FUNCTION "FC_CLEAN_ROOM" : VOID
TITLE =FC CLEAN ROOM
{ S7_language := '9(1) Angielski (Stany Zjednoczone)  11.01.2022  09:45:15' }
VERSION : 0.1


VAR_TEMP
  PREHEATING_TIME_SP : S5TIME ;
  FOLLOW_UP_PURGING_ON : BOOL ;
  PREPURING_ON : BOOL ;
  CR_HUM_RELEASE : BOOL ;
  F_UP_PURGING_TIME_SP : S5TIME ;
  H_84CLM82_HUM_SWP : REAL ;
  H_84CLM82_DEHUM_SWP : REAL ;
  T_84CLT81_COOL_SWP : REAL ;
  T_84CLT81_HEAT_SWP : REAL ;
  H_84CLM82_READY_LOW : REAL ;
  H_84CLM82_READY_HIGH : REAL ;
  T_84CLT81_READY_LOW : REAL ;
  T_84CLT81_READY_HIGH : REAL ;
  T_81CLM10_HUM_SP : REAL ;
  T_81CLM10_HUM_AV_REL : REAL ;
  T_81CLM10_HUM_SP_DINT : DINT ;
  T_84CLT32_COOL_SWP : REAL ;
  T_84CLT32_HEAT_SWP : REAL ;
  T_AV_REAL : REAL ;
  T_AV_DINT : DINT ;
END_VAR
BEGIN
NETWORK
TITLE =CLEAN ROOM ON
//********************************************************************************
//
//                         CLEAN ROOM START / STOP
//
//********************************************************************************
//
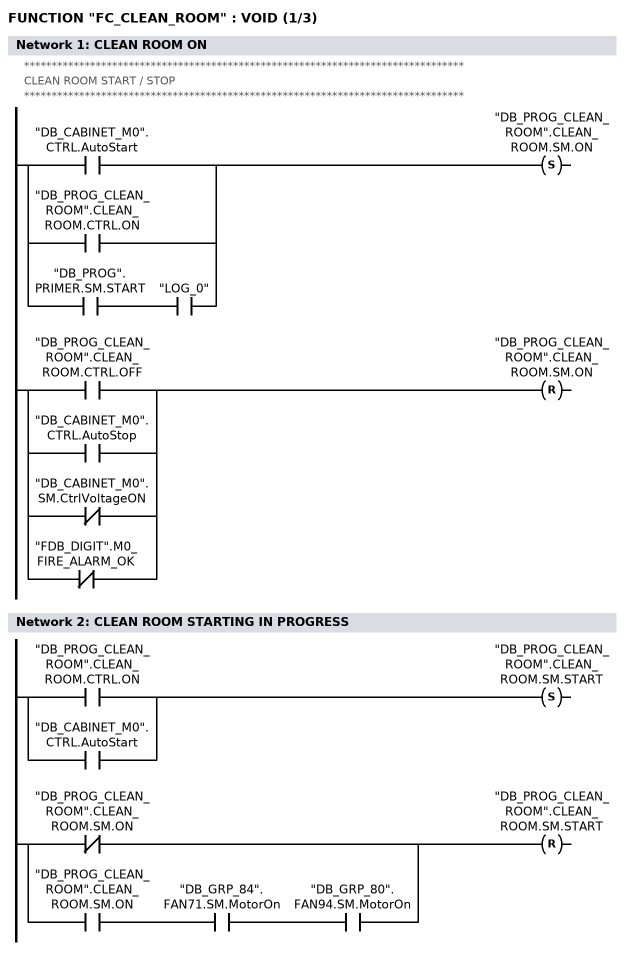
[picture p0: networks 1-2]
      U(    ;
      O     "DB_CABINET_M0".CTRL.AutoStart;
      O     "DB_PROG_CLEAN_ROOM".CLEAN_ROOM.CTRL.ON;
      O     ;
      U     "DB_PROG".PRIMER.SM.START;
      U     "LOG_0";
      )     ;
      S     "DB_PROG_CLEAN_ROOM".CLEAN_ROOM.SM.ON;
      U(    ;
      O     "DB_PROG_CLEAN_ROOM".CLEAN_ROOM.CTRL.OFF;
      O     "DB_CABINET_M0".CTRL.AutoStop;
      ON    "DB_CABINET_M0".SM.CtrlVoltageON;
      ON    "FDB_DIGIT".M0_FIRE_ALARM_OK;
      )     ;
      R     "DB_PROG_CLEAN_ROOM".CLEAN_ROOM.SM.ON;
      NOP   0;
NETWORK
TITLE =CLEAN ROOM STARTING IN PROGRESS

      U(    ;
      O     "DB_PROG_CLEAN_ROOM".CLEAN_ROOM.CTRL.ON;
      O     "DB_CABINET_M0".CTRL.AutoStart;
      )     ;
      S     "DB_PROG_CLEAN_ROOM".CLEAN_ROOM.SM.START;
      U(    ;
      ON    "DB_PROG_CLEAN_ROOM".CLEAN_ROOM.SM.ON;
      O     ;
      U     "DB_PROG_CLEAN_ROOM".CLEAN_ROOM.SM.ON;
      U     "DB_GRP_84".FAN71.SM.MotorOn;
      U     "DB_GRP_80".FAN94.SM.MotorOn;
      )     ;
      R     "DB_PROG_CLEAN_ROOM".CLEAN_ROOM.SM.START;
      NOP   0;
NETWORK
TITLE =CLEAN ROOM STOPPING IN PROGRESS
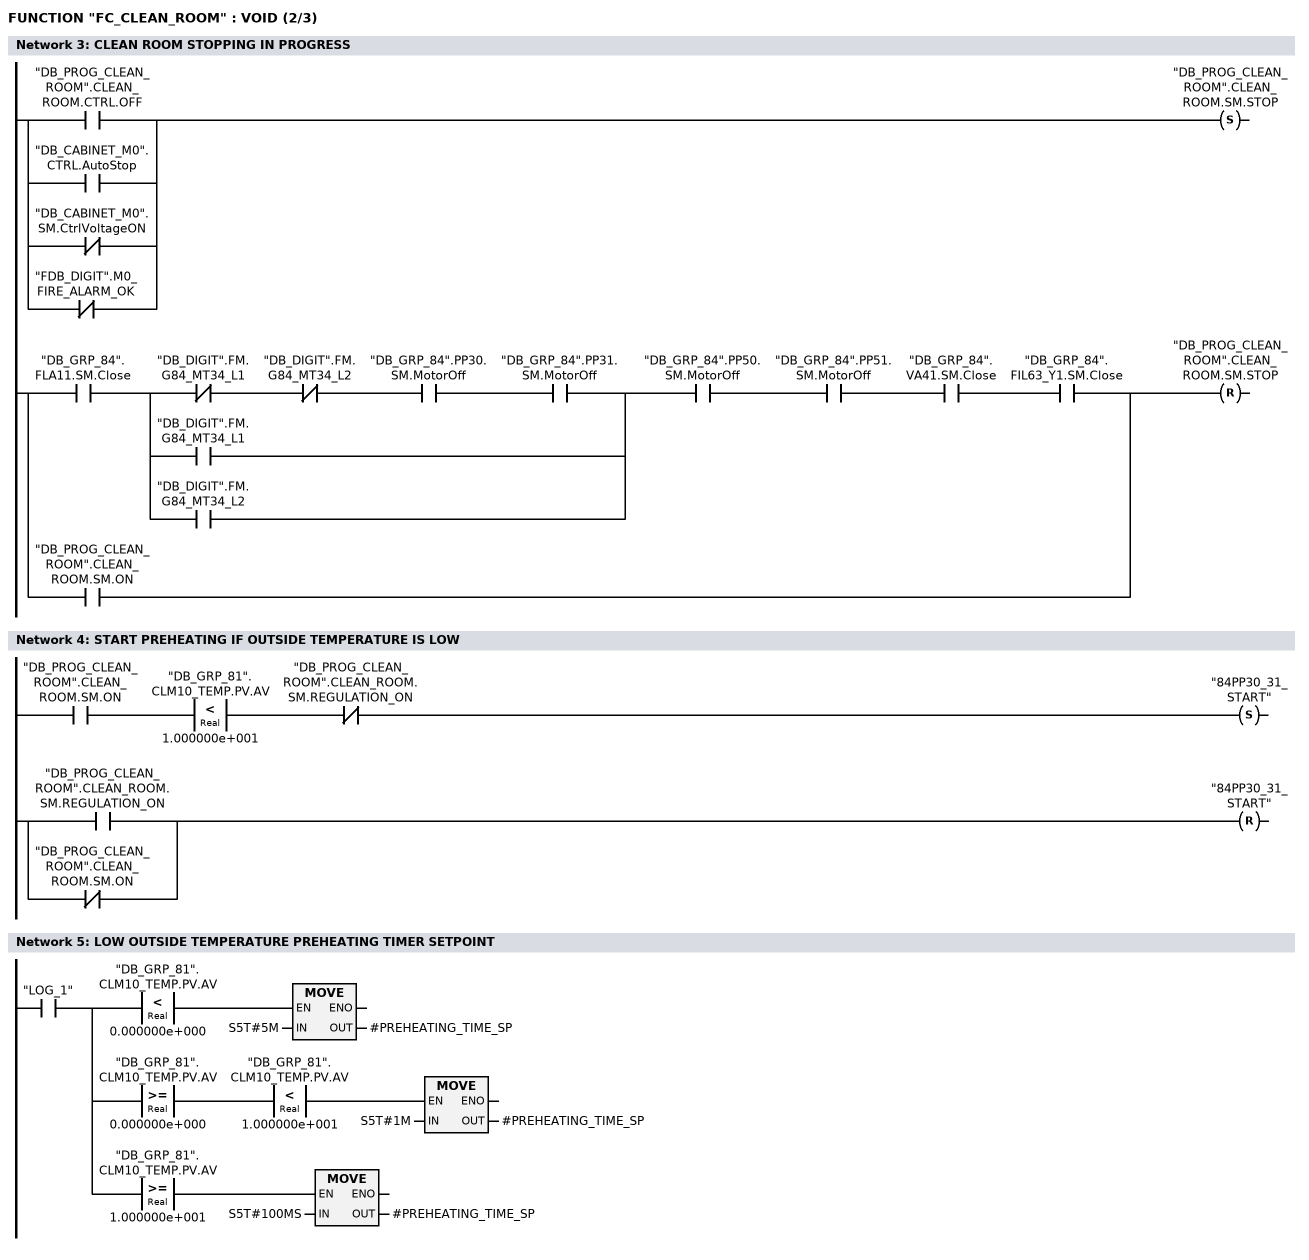
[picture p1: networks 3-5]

      U(    ;
      O     "DB_PROG_CLEAN_ROOM".CLEAN_ROOM.CTRL.OFF;
      O     "DB_CABINET_M0".CTRL.AutoStop;
      ON    "DB_CABINET_M0".SM.CtrlVoltageON;
      ON    "FDB_DIGIT".M0_FIRE_ALARM_OK;
      )     ;
      S     "DB_PROG_CLEAN_ROOM".CLEAN_ROOM.SM.STOP;
      U(    ;
      U     "DB_GRP_84".FLA11.SM.Close;
      U(    ;
      UN    "DB_DIGIT".FM.G84_MT34_L1;
      UN    "DB_DIGIT".FM.G84_MT34_L2;
      U     "DB_GRP_84".PP30.SM.MotorOff;
      U     "DB_GRP_84".PP31.SM.MotorOff;
      O     "DB_DIGIT".FM.G84_MT34_L1;
      O     "DB_DIGIT".FM.G84_MT34_L2;
      )     ;
      U     "DB_GRP_84".PP50.SM.MotorOff;
      U     "DB_GRP_84".PP51.SM.MotorOff;
      U     "DB_GRP_84".VA41.SM.Close;
      U     "DB_GRP_84".FIL63_Y1.SM.Close;
      O     "DB_PROG_CLEAN_ROOM".CLEAN_ROOM.SM.ON;
      )     ;
      R     "DB_PROG_CLEAN_ROOM".CLEAN_ROOM.SM.STOP;
      NOP   0;
NETWORK
TITLE =START PREHEATING IF OUTSIDE TEMPERATURE IS LOW

      U     "DB_PROG_CLEAN_ROOM".CLEAN_ROOM.SM.ON;
      U(    ;
      L     "DB_GRP_81".CLM10_TEMP.PV.AV;
      L     1.000000e+001;
      <R    ;
      )     ;
      UN    "DB_PROG_CLEAN_ROOM".CLEAN_ROOM.SM.REGULATION_ON;
      S     "84PP30_31_START";
      U(    ;
      O     "DB_PROG_CLEAN_ROOM".CLEAN_ROOM.SM.REGULATION_ON;
      ON    "DB_PROG_CLEAN_ROOM".CLEAN_ROOM.SM.ON;
      )     ;
      R     "84PP30_31_START";
      NOP   0;
NETWORK
TITLE =LOW OUTSIDE TEMPERATURE PREHEATING TIMER SETPOINT

      U     "LOG_1";
      =     L     66.0;
      U     L     66.0;
      U(    ;
      L     "DB_GRP_81".CLM10_TEMP.PV.AV;
      L     0.000000e+000;
      <R    ;
      )     ;
      SPBNB _001;
      L     S5T#5M;
      T     #PREHEATING_TIME_SP;
_001: NOP   0;
      U     L     66.0;
      U(    ;
      L     "DB_GRP_81".CLM10_TEMP.PV.AV;
      L     0.000000e+000;
      >=R   ;
      )     ;
      U(    ;
      L     "DB_GRP_81".CLM10_TEMP.PV.AV;
      L     1.000000e+001;
      <R    ;
      )     ;
      SPBNB _002;
      L     S5T#1M;
      T     #PREHEATING_TIME_SP;
_002: NOP   0;
      U     L     66.0;
      U(    ;
      L     "DB_GRP_81".CLM10_TEMP.PV.AV;
      L     1.000000e+001;
      >=R   ;
      )     ;
      SPBNB _003;
      L     S5T#100MS;
      T     #PREHEATING_TIME_SP;
_003: NOP   0;
NETWORK
TITLE =LOW OUTSIDE TEMPERATURE PREHEATING TIMER
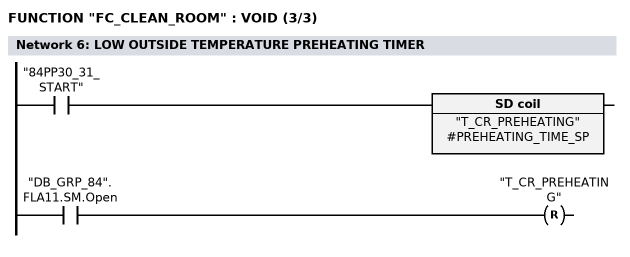
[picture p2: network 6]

      U     "84PP30_31_START";
      L     #PREHEATING_TIME_SP;
      SE    "T_CR_PREHEATING";
      U     "DB_GRP_84".FLA11.SM.Open;
      R     "T_CR_PREHEATING";
      NOP   0;
      NOP   0;
      NOP   0;
NETWORK
TITLE =OPEN AIR SUPPLY UNIT FLAP

      U(    ;
      U     "84PP30_31_START";
      U     "T_CR_PREHEATING";
      O(    ;
      UN    "84PP30_31_START";
      L     S5T#100MS;
      SE    "T_CR_ASU_FLAPS_OPEN_DEL";
      NOP   0;
      NOP   0;
      NOP   0;
      U     "T_CR_ASU_FLAPS_OPEN_DEL";
      )     ;
      )     ;
      U     "DB_PROG_CLEAN_ROOM".CLEAN_ROOM.SM.ON;
      =     "CR_OPEN_ASU_FLAP";
NETWORK
TITLE =CLOSE AIR SUPPLY UNIT FLAP
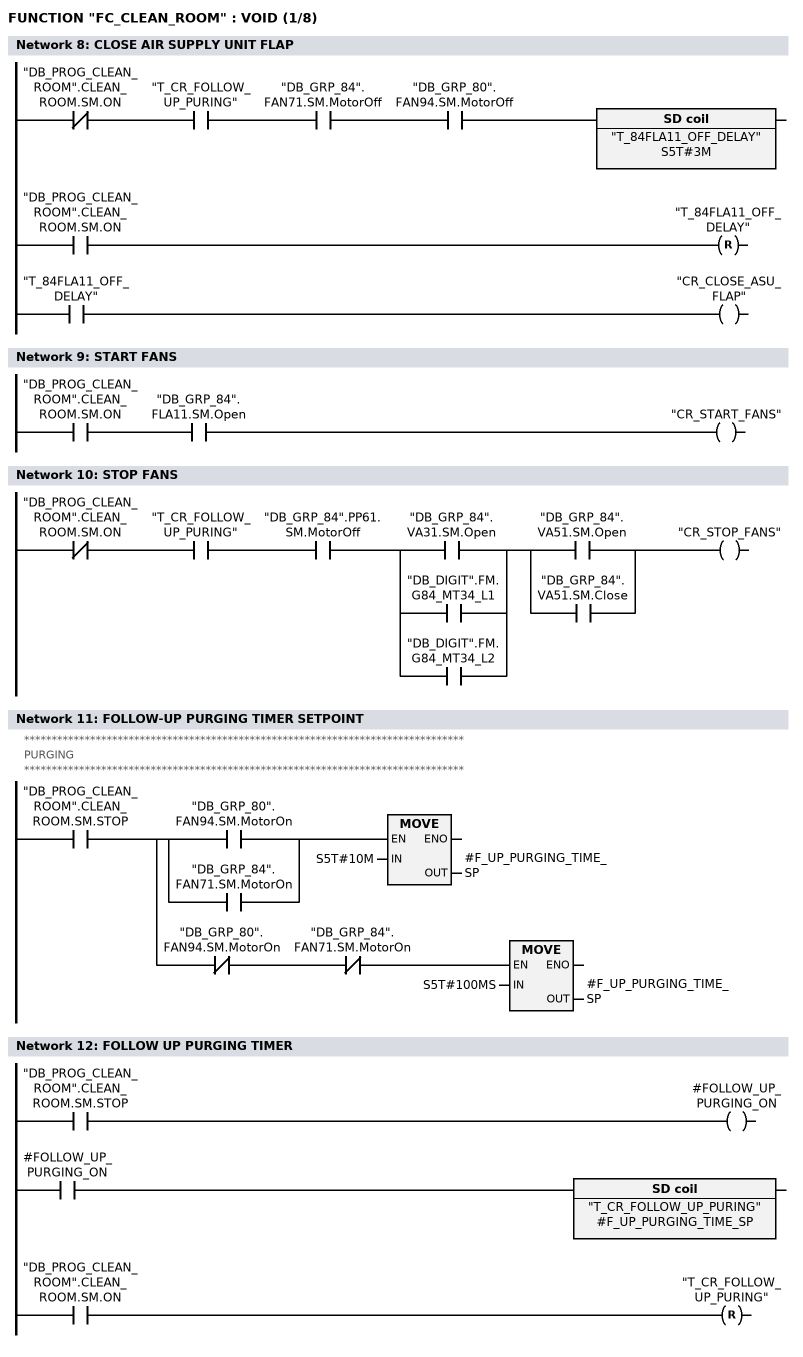
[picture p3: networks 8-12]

      UN    "DB_PROG_CLEAN_ROOM".CLEAN_ROOM.SM.ON;
      U     "T_CR_FOLLOW_UP_PURING";
      U     "DB_GRP_84".FAN71.SM.MotorOff;
      U     "DB_GRP_80".FAN94.SM.MotorOff;
      L     S5T#3M;
      SE    "T_84FLA11_OFF_DELAY";
      U     "DB_PROG_CLEAN_ROOM".CLEAN_ROOM.SM.ON;
      R     "T_84FLA11_OFF_DELAY";
      NOP   0;
      NOP   0;
      U     "T_84FLA11_OFF_DELAY";
      =     "CR_CLOSE_ASU_FLAP";
NETWORK
TITLE =START FANS

      U     "DB_PROG_CLEAN_ROOM".CLEAN_ROOM.SM.ON;
      U     "DB_GRP_84".FLA11.SM.Open;
      =     "CR_START_FANS";
NETWORK
TITLE =STOP FANS

      UN    "DB_PROG_CLEAN_ROOM".CLEAN_ROOM.SM.ON;
      U     "T_CR_FOLLOW_UP_PURING";
      U     "DB_GRP_84".PP61.SM.MotorOff;
      U(    ;
      O     "DB_GRP_84".VA31.SM.Open;
      O     "DB_DIGIT".FM.G84_MT34_L1;
      O     "DB_DIGIT".FM.G84_MT34_L2;
      )     ;
      U(    ;
      O     "DB_GRP_84".VA51.SM.Open;
      O     "DB_GRP_84".VA51.SM.Close;
      )     ;
      =     "CR_STOP_FANS";
NETWORK
TITLE =FOLLOW-UP PURGING TIMER SETPOINT
//********************************************************************************
//
//                                   PURGING
//
//********************************************************************************
//
      U     "DB_PROG_CLEAN_ROOM".CLEAN_ROOM.SM.STOP;
      =     L     66.0;
      U     L     66.0;
      U(    ;
      O     "DB_GRP_80".FAN94.SM.MotorOn;
      O     "DB_GRP_84".FAN71.SM.MotorOn;
      )     ;
      SPBNB _004;
      L     S5T#10M;
      T     #F_UP_PURGING_TIME_SP;
_004: NOP   0;
      U     L     66.0;
      UN    "DB_GRP_80".FAN94.SM.MotorOn;
      UN    "DB_GRP_84".FAN71.SM.MotorOn;
      SPBNB _005;
      L     S5T#100MS;
      T     #F_UP_PURGING_TIME_SP;
_005: NOP   0;
NETWORK
TITLE =FOLLOW UP PURGING TIMER

      U     "DB_PROG_CLEAN_ROOM".CLEAN_ROOM.SM.STOP;
      =     #FOLLOW_UP_PURGING_ON;
      U     #FOLLOW_UP_PURGING_ON;
      L     #F_UP_PURGING_TIME_SP;
      SE    "T_CR_FOLLOW_UP_PURING";
      U     "DB_PROG_CLEAN_ROOM".CLEAN_ROOM.SM.ON;
      R     "T_CR_FOLLOW_UP_PURING";
      NOP   0;
      NOP   0;
      NOP   0;
NETWORK
TITLE =FOLLOW-UP PURGING TIMER RUNNING
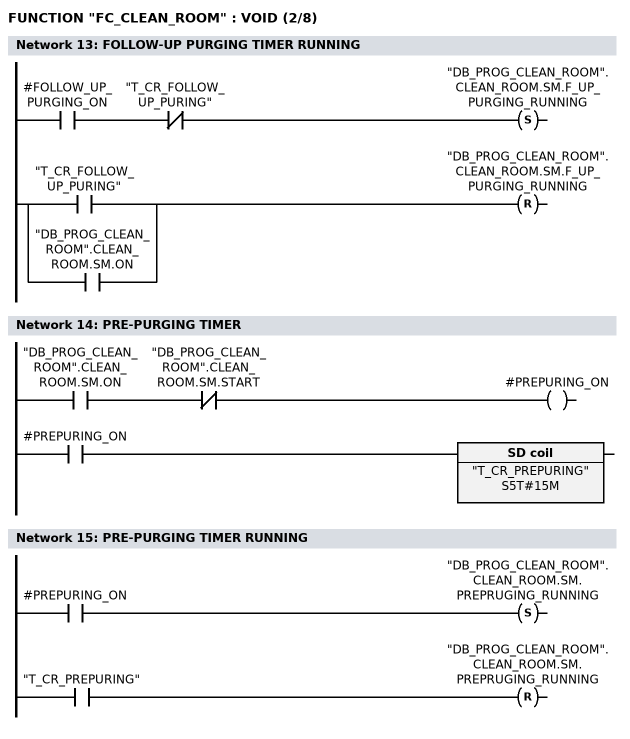
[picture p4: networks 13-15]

      U     #FOLLOW_UP_PURGING_ON;
      UN    "T_CR_FOLLOW_UP_PURING";
      S     "DB_PROG_CLEAN_ROOM".CLEAN_ROOM.SM.F_UP_PURGING_RUNNING;
      U(    ;
      O     "T_CR_FOLLOW_UP_PURING";
      O     "DB_PROG_CLEAN_ROOM".CLEAN_ROOM.SM.ON;
      )     ;
      R     "DB_PROG_CLEAN_ROOM".CLEAN_ROOM.SM.F_UP_PURGING_RUNNING;
      NOP   0;
NETWORK
TITLE =PRE-PURGING TIMER

      U     "DB_PROG_CLEAN_ROOM".CLEAN_ROOM.SM.ON;
      UN    "DB_PROG_CLEAN_ROOM".CLEAN_ROOM.SM.START;
      =     #PREPURING_ON;
      U     #PREPURING_ON;
      L     S5T#15M;
      SE    "T_CR_PREPURING";
      NOP   0;
      NOP   0;
      NOP   0;
      NOP   0;
NETWORK
TITLE =PRE-PURGING TIMER RUNNING

      U     #PREPURING_ON;
      S     "DB_PROG_CLEAN_ROOM".CLEAN_ROOM.SM.PREPRUGING_RUNNING;
      U     "T_CR_PREPURING";
      R     "DB_PROG_CLEAN_ROOM".CLEAN_ROOM.SM.PREPRUGING_RUNNING;
      NOP   0;
NETWORK
TITLE =AIR SUPPLY UNIT REGULATION ON
//********************************************************************************
//
//                           AIR SUPPLY UNIT REGULATION
//
//********************************************************************************
//
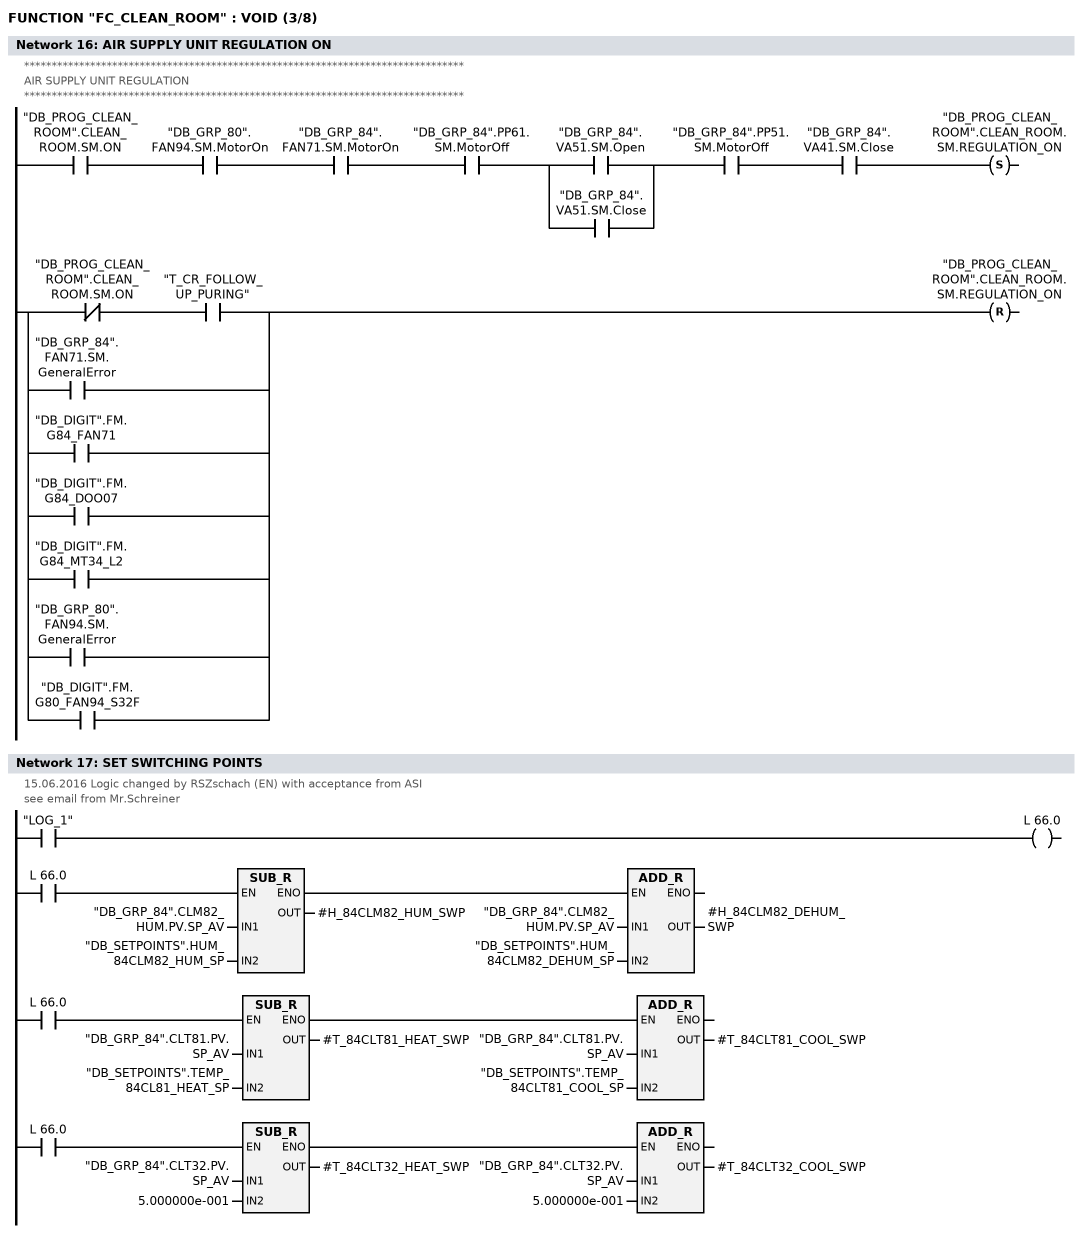
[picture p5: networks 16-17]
      U     "DB_PROG_CLEAN_ROOM".CLEAN_ROOM.SM.ON;
      U     "DB_GRP_80".FAN94.SM.MotorOn;
      U     "DB_GRP_84".FAN71.SM.MotorOn;
      U     "DB_GRP_84".PP61.SM.MotorOff;
      U(    ;
      O     "DB_GRP_84".VA51.SM.Open;
      O     "DB_GRP_84".VA51.SM.Close;
      )     ;
      U     "DB_GRP_84".PP51.SM.MotorOff;
      U     "DB_GRP_84".VA41.SM.Close;
      S     "DB_PROG_CLEAN_ROOM".CLEAN_ROOM.SM.REGULATION_ON;
      U(    ;
      UN    "DB_PROG_CLEAN_ROOM".CLEAN_ROOM.SM.ON;
      U     "T_CR_FOLLOW_UP_PURING";
      O     "DB_GRP_84".FAN71.SM.GeneralError;
      O     "DB_DIGIT".FM.G84_FAN71;
      O     "DB_DIGIT".FM.G84_DOO07;
      O     "DB_DIGIT".FM.G84_MT34_L2;
      O     "DB_GRP_80".FAN94.SM.GeneralError;
      O     "DB_DIGIT".FM.G80_FAN94_S32F;
      )     ;
      R     "DB_PROG_CLEAN_ROOM".CLEAN_ROOM.SM.REGULATION_ON;
      NOP   0;
NETWORK
TITLE =SET SWITCHING POINTS
//15.06.2016 Logic changed by RSZschach (EN) with acceptance from ASI
//see email from Mr.Schreiner
      U     "LOG_1";
      =     L     66.0;
      U(    ;
      U     L     66.0;
      SPBNB _006;
      L     "DB_GRP_84".CLM82_HUM.PV.SP_AV;
      L     "DB_SETPOINTS".HUM_84CLM82_HUM_SP;
      -R    ;
      T     #H_84CLM82_HUM_SWP;
      UN    OV;
      SAVE  ;
      CLR   ;
_006: U     BIE;
      )     ;
      SPBNB _007;
      L     "DB_GRP_84".CLM82_HUM.PV.SP_AV;
      L     "DB_SETPOINTS".HUM_84CLM82_DEHUM_SP;
      +R    ;
      T     #H_84CLM82_DEHUM_SWP;
_007: NOP   0;
      U(    ;
      U     L     66.0;
      SPBNB _008;
      L     "DB_GRP_84".CLT81.PV.SP_AV;
      L     "DB_SETPOINTS".TEMP_84CL81_HEAT_SP;
      -R    ;
      T     #T_84CLT81_HEAT_SWP;
      UN    OV;
      SAVE  ;
      CLR   ;
_008: U     BIE;
      )     ;
      SPBNB _009;
      L     "DB_GRP_84".CLT81.PV.SP_AV;
      L     "DB_SETPOINTS".TEMP_84CLT81_COOL_SP;
      +R    ;
      T     #T_84CLT81_COOL_SWP;
_009: NOP   0;
      U(    ;
      U     L     66.0;
      SPBNB _00a;
      L     "DB_GRP_84".CLT32.PV.SP_AV;
      L     5.000000e-001;
      -R    ;
      T     #T_84CLT32_HEAT_SWP;
      UN    OV;
      SAVE  ;
      CLR   ;
_00a: U     BIE;
      )     ;
      SPBNB _00b;
      L     "DB_GRP_84".CLT32.PV.SP_AV;
      L     5.000000e-001;
      +R    ;
      T     #T_84CLT32_COOL_SWP;
_00b: NOP   0;
NETWORK
TITLE =AIR SUPPLY UNIT CONTROL LOOP CASE/CONDITION 1
//15.06.2016 Logic changed by RSZschach (EN) with acceptance from ASI
//see email from Mr.Schreiner
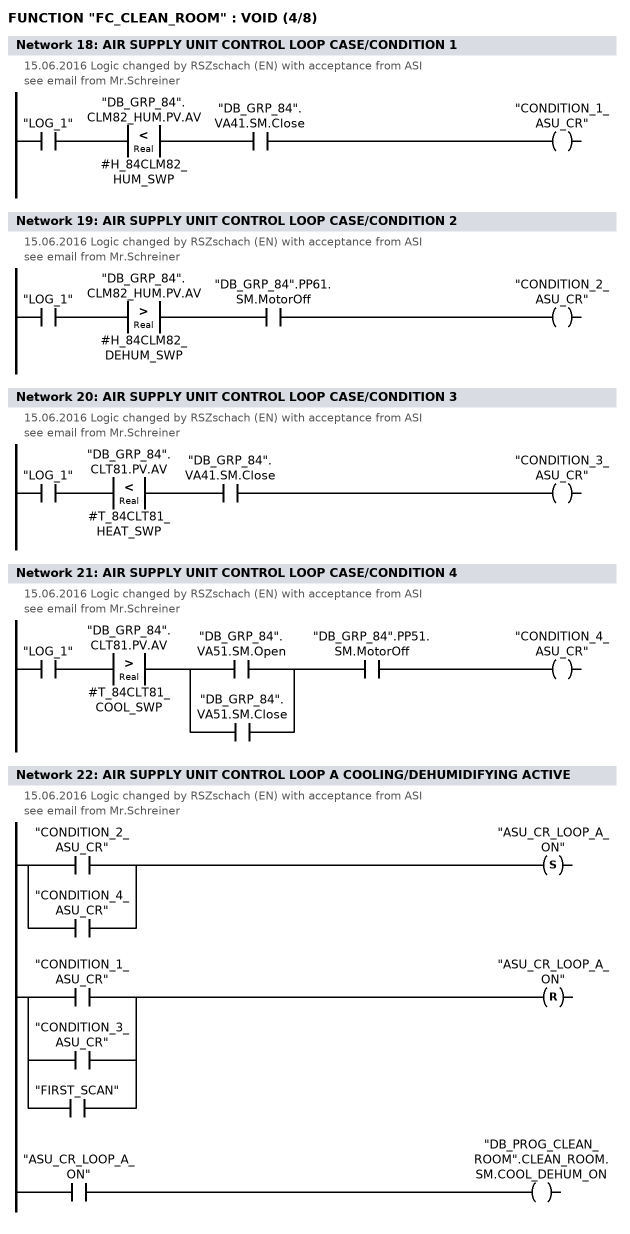
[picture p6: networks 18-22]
      U     "LOG_1";
      U(    ;
      L     "DB_GRP_84".CLM82_HUM.PV.AV;
      L     #H_84CLM82_HUM_SWP;
      <R    ;
      )     ;
      U     "DB_GRP_84".VA41.SM.Close;
      =     "CONDITION_1_ASU_CR";
NETWORK
TITLE =AIR SUPPLY UNIT CONTROL LOOP CASE/CONDITION 2
//15.06.2016 Logic changed by RSZschach (EN) with acceptance from ASI
//see email from Mr.Schreiner
      U     "LOG_1";
      U(    ;
      L     "DB_GRP_84".CLM82_HUM.PV.AV;
      L     #H_84CLM82_DEHUM_SWP;
      >R    ;
      )     ;
      U     "DB_GRP_84".PP61.SM.MotorOff;
      =     "CONDITION_2_ASU_CR";
NETWORK
TITLE =AIR SUPPLY UNIT CONTROL LOOP CASE/CONDITION 3
//15.06.2016 Logic changed by RSZschach (EN) with acceptance from ASI
//see email from Mr.Schreiner
      U     "LOG_1";
      U(    ;
      L     "DB_GRP_84".CLT81.PV.AV;
      L     #T_84CLT81_HEAT_SWP;
      <R    ;
      )     ;
      U     "DB_GRP_84".VA41.SM.Close;
      =     "CONDITION_3_ASU_CR";
NETWORK
TITLE =AIR SUPPLY UNIT CONTROL LOOP CASE/CONDITION 4
//15.06.2016 Logic changed by RSZschach (EN) with acceptance from ASI
//see email from Mr.Schreiner
      U     "LOG_1";
      U(    ;
      L     "DB_GRP_84".CLT81.PV.AV;
      L     #T_84CLT81_COOL_SWP;
      >R    ;
      )     ;
      U(    ;
      O     "DB_GRP_84".VA51.SM.Open;
      O     "DB_GRP_84".VA51.SM.Close;
      )     ;
      U     "DB_GRP_84".PP51.SM.MotorOff;
      =     "CONDITION_4_ASU_CR";
NETWORK
TITLE =AIR SUPPLY UNIT CONTROL LOOP A COOLING/DEHUMIDIFYING ACTIVE
//15.06.2016 Logic changed by RSZschach (EN) with acceptance from ASI
//see email from Mr.Schreiner
      U(    ;
      O     "CONDITION_2_ASU_CR";
      O     "CONDITION_4_ASU_CR";
      )     ;
      S     "ASU_CR_LOOP_A_ON";
      U(    ;
      O     "CONDITION_1_ASU_CR";
      O     "CONDITION_3_ASU_CR";
      O     "FIRST_SCAN";
      )     ;
      R     "ASU_CR_LOOP_A_ON";
      U     "ASU_CR_LOOP_A_ON";
      =     "DB_PROG_CLEAN_ROOM".CLEAN_ROOM.SM.COOL_DEHUM_ON;
NETWORK
TITLE =AIR SUPPLY UNIT CONTROL LOOP B HUMIDIFYING ACTIVE
//15.06.2016 Logic changed by RSZschach (EN) with acceptance from ASI
//see email from Mr.Schreiner
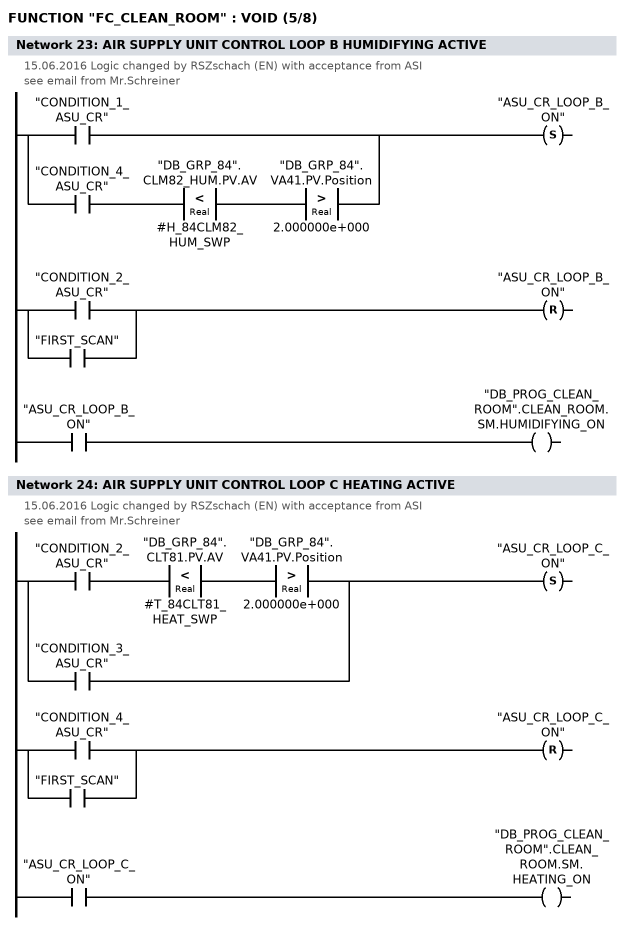
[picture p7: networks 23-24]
      U(    ;
      O     "CONDITION_1_ASU_CR";
      O     ;
      U     "CONDITION_4_ASU_CR";
      U(    ;
      L     "DB_GRP_84".CLM82_HUM.PV.AV;
      L     #H_84CLM82_HUM_SWP;
      <R    ;
      )     ;
      U(    ;
      L     "DB_GRP_84".VA41.PV.Position;
      L     2.000000e+000;
      >R    ;
      )     ;
      )     ;
      S     "ASU_CR_LOOP_B_ON";
      U(    ;
      O     "CONDITION_2_ASU_CR";
      O     "FIRST_SCAN";
      )     ;
      R     "ASU_CR_LOOP_B_ON";
      U     "ASU_CR_LOOP_B_ON";
      =     "DB_PROG_CLEAN_ROOM".CLEAN_ROOM.SM.HUMIDIFYING_ON;
NETWORK
TITLE =AIR SUPPLY UNIT CONTROL LOOP C HEATING ACTIVE
//15.06.2016 Logic changed by RSZschach (EN) with acceptance from ASI
//see email from Mr.Schreiner
      U(    ;
      U     "CONDITION_2_ASU_CR";
      U(    ;
      L     "DB_GRP_84".CLT81.PV.AV;
      L     #T_84CLT81_HEAT_SWP;
      <R    ;
      )     ;
      U(    ;
      L     "DB_GRP_84".VA41.PV.Position;
      L     2.000000e+000;
      >R    ;
      )     ;
      O     "CONDITION_3_ASU_CR";
      )     ;
      S     "ASU_CR_LOOP_C_ON";
      U(    ;
      O     "CONDITION_4_ASU_CR";
      O     "FIRST_SCAN";
      )     ;
      R     "ASU_CR_LOOP_C_ON";
      U     "ASU_CR_LOOP_C_ON";
      =     "DB_PROG_CLEAN_ROOM".CLEAN_ROOM.SM.HEATING_ON;
NETWORK
TITLE =AIR SUPPLY UNIT CONTROL LOOP D PREHEATING ACTIVE
//15.06.2016 Logic changed by RSZschach (EN) with acceptance from ASI
//see email from Mr.Schreiner
//
//#T_84CLT32_HEAT_SWP
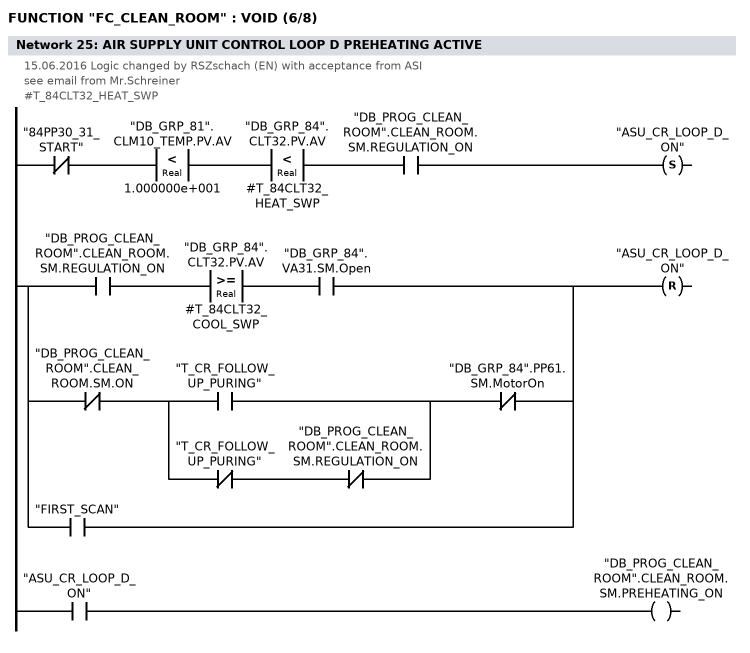
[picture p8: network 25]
      UN    "84PP30_31_START";
      U(    ;
      L     "DB_GRP_81".CLM10_TEMP.PV.AV;
      L     1.000000e+001;
      <R    ;
      )     ;
      U(    ;
      L     "DB_GRP_84".CLT32.PV.AV;
      L     #T_84CLT32_HEAT_SWP;
      <R    ;
      )     ;
      U     "DB_PROG_CLEAN_ROOM".CLEAN_ROOM.SM.REGULATION_ON;
      S     "ASU_CR_LOOP_D_ON";
      U(    ;
      U     "DB_PROG_CLEAN_ROOM".CLEAN_ROOM.SM.REGULATION_ON;
      U(    ;
      L     "DB_GRP_84".CLT32.PV.AV;
      L     #T_84CLT32_COOL_SWP;
      >=R   ;
      )     ;
      U     "DB_GRP_84".VA31.SM.Open;
      O     ;
      UN    "DB_PROG_CLEAN_ROOM".CLEAN_ROOM.SM.ON;
      U(    ;
      O     "T_CR_FOLLOW_UP_PURING";
      O     ;
      UN    "T_CR_FOLLOW_UP_PURING";
      UN    "DB_PROG_CLEAN_ROOM".CLEAN_ROOM.SM.REGULATION_ON;
      )     ;
      UN    "DB_GRP_84".PP61.SM.MotorOn;
      O     "FIRST_SCAN";
      )     ;
      R     "ASU_CR_LOOP_D_ON";
      U     "ASU_CR_LOOP_D_ON";
      =     "DB_PROG_CLEAN_ROOM".CLEAN_ROOM.SM.PREHEATING_ON;
NETWORK
TITLE =PROCESS CONDITIONS - TEMPERATURE AND HUMIDITY
//********************************************************************************
//
//                              PROCESS CONDITIONS
//
//********************************************************************************
//15.06.2016 Logic changed by RSZschach (EN) with acceptance from ASI
//see email from Mr.Schreiner
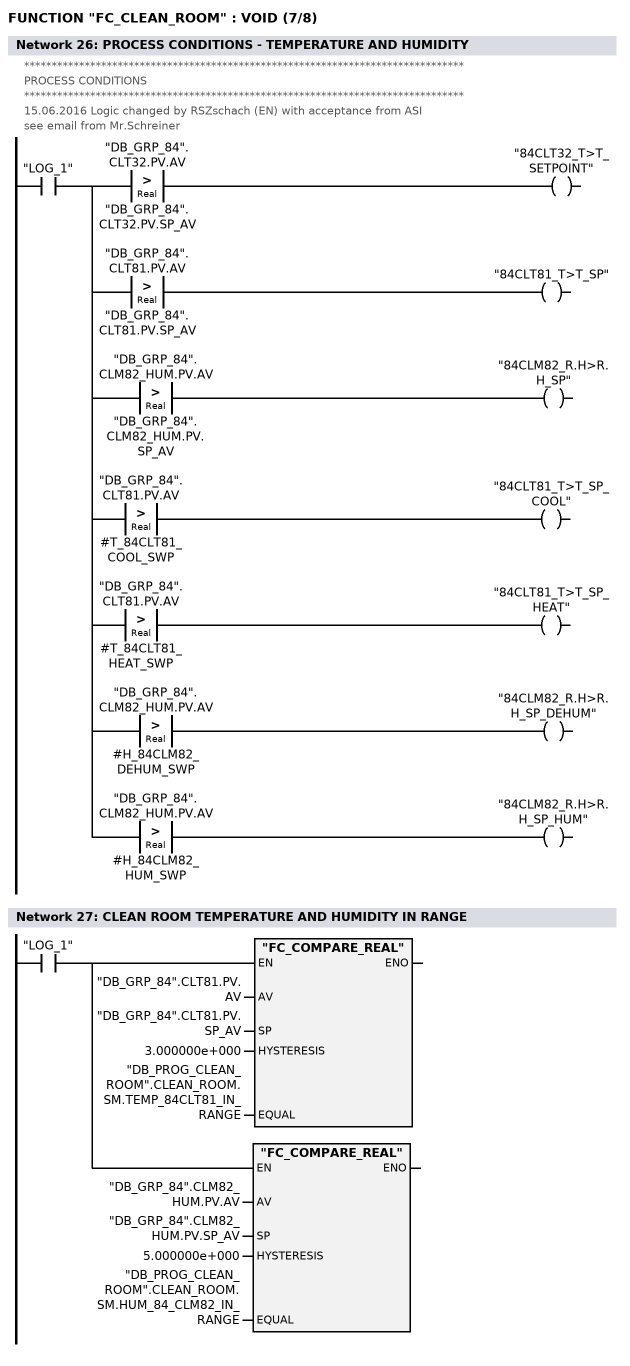
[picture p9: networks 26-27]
      U     "LOG_1";
      =     L     66.0;
      U     L     66.0;
      U(    ;
      L     "DB_GRP_84".CLT32.PV.AV;
      L     "DB_GRP_84".CLT32.PV.SP_AV;
      >R    ;
      )     ;
      =     "84CLT32_T>T_SETPOINT";
      U     L     66.0;
      U(    ;
      L     "DB_GRP_84".CLT81.PV.AV;
      L     "DB_GRP_84".CLT81.PV.SP_AV;
      >R    ;
      )     ;
      =     "84CLT81_T>T_SP";
      U     L     66.0;
      U(    ;
      L     "DB_GRP_84".CLM82_HUM.PV.AV;
      L     "DB_GRP_84".CLM82_HUM.PV.SP_AV;
      >R    ;
      )     ;
      =     "84CLM82_R.H>R.H_SP";
      U     L     66.0;
      U(    ;
      L     "DB_GRP_84".CLT81.PV.AV;
      L     #T_84CLT81_COOL_SWP;
      >R    ;
      )     ;
      =     "84CLT81_T>T_SP_COOL";
      U     L     66.0;
      U(    ;
      L     "DB_GRP_84".CLT81.PV.AV;
      L     #T_84CLT81_HEAT_SWP;
      >R    ;
      )     ;
      =     "84CLT81_T>T_SP_HEAT";
      U     L     66.0;
      U(    ;
      L     "DB_GRP_84".CLM82_HUM.PV.AV;
      L     #H_84CLM82_DEHUM_SWP;
      >R    ;
      )     ;
      =     "84CLM82_R.H>R.H_SP_DEHUM";
      U     L     66.0;
      U(    ;
      L     "DB_GRP_84".CLM82_HUM.PV.AV;
      L     #H_84CLM82_HUM_SWP;
      >R    ;
      )     ;
      =     "84CLM82_R.H>R.H_SP_HUM";
NETWORK
TITLE =CLEAN ROOM TEMPERATURE AND HUMIDITY IN RANGE

      U     "LOG_1";
      =     L     66.0;
      U     L     66.0;
      SPBNB _00c;
      CALL "FC_COMPARE_REAL" (
           AV                       := "DB_GRP_84".CLT81.PV.AV,
           SP                       := "DB_GRP_84".CLT81.PV.SP_AV,
           HYSTERESIS               := 3.000000e+000,
           EQUAL                    := "DB_PROG_CLEAN_ROOM".CLEAN_ROOM.SM.TEMP_84CLT81_IN_RANGE);
_00c: NOP   0;
      U     L     66.0;
      SPBNB _00d;
      CALL "FC_COMPARE_REAL" (
           AV                       := "DB_GRP_84".CLM82_HUM.PV.AV,
           SP                       := "DB_GRP_84".CLM82_HUM.PV.SP_AV,
           HYSTERESIS               := 5.000000e+000,
           EQUAL                    := "DB_PROG_CLEAN_ROOM".CLEAN_ROOM.SM.HUM_84_CLM82_IN_RANGE);
_00d: NOP   0;
NETWORK
TITLE =WINDOW FOR READY STATUS IN POWER SAVING MODE 2
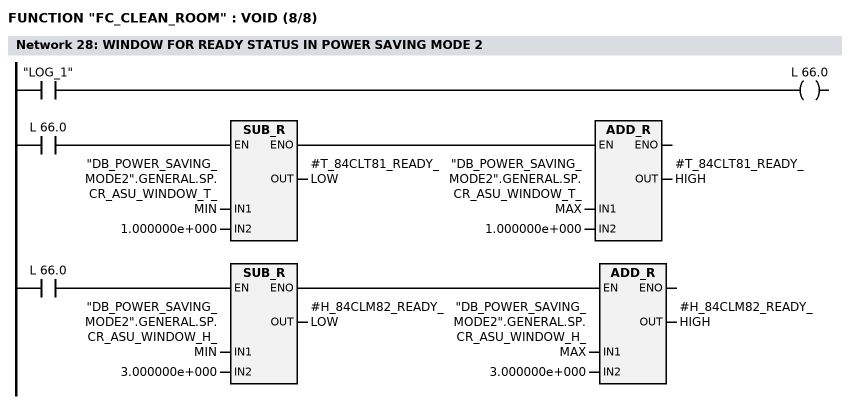
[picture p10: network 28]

      U     "LOG_1";
      =     L     66.0;
      U(    ;
      U     L     66.0;
      SPBNB _00e;
      L     "DB_POWER_SAVING_MODE2".GENERAL.SP.CR_ASU_WINDOW_T_MIN;
      L     1.000000e+000;
      -R    ;
      T     #T_84CLT81_READY_LOW;
      UN    OV;
      SAVE  ;
      CLR   ;
_00e: U     BIE;
      )     ;
      SPBNB _00f;
      L     "DB_POWER_SAVING_MODE2".GENERAL.SP.CR_ASU_WINDOW_T_MAX;
      L     1.000000e+000;
      +R    ;
      T     #T_84CLT81_READY_HIGH;
_00f: NOP   0;
      U(    ;
      U     L     66.0;
      SPBNB _010;
      L     "DB_POWER_SAVING_MODE2".GENERAL.SP.CR_ASU_WINDOW_H_MIN;
      L     3.000000e+000;
      -R    ;
      T     #H_84CLM82_READY_LOW;
      UN    OV;
      SAVE  ;
      CLR   ;
_010: U     BIE;
      )     ;
      SPBNB _011;
      L     "DB_POWER_SAVING_MODE2".GENERAL.SP.CR_ASU_WINDOW_H_MAX;
      L     3.000000e+000;
      +R    ;
      T     #H_84CLM82_READY_HIGH;
_011: NOP   0;
NETWORK
TITLE =CLEAN ROOM READY - TEMPERATURE AND HUMIDITY IN RANGE
//********************************************************************************
//
//                                CLEAN ROOM READY
//
//********************************************************************************
//
      U(    ;
      U     "DB_PROG_CLEAN_ROOM".CLEAN_ROOM.SM.ON;
      UN    "DB_PROG_CLEAN_ROOM".CLEAN_ROOM.SM.START;
      U     "T_CR_PREPURING";
      U(    ;
      UN    "DB_POWER_SAVING_MODE2".GENERAL.SM.CR_MODE_2_ON;
      U     "DB_PROG_CLEAN_ROOM".CLEAN_ROOM.SM.TEMP_84CLT81_IN_RANGE;
      U     "DB_PROG_CLEAN_ROOM".CLEAN_ROOM.SM.HUM_84_CLM82_IN_RANGE;
      O     ;
      U     "DB_POWER_SAVING_MODE2".GENERAL.SM.CR_MODE_2_ON;
      U(    ;
      L     "DB_GRP_84".CLT81.PV.AV;
      L     #T_84CLT81_READY_LOW;
      >=R   ;
      )     ;
      U(    ;
      L     "DB_GRP_84".CLT81.PV.AV;
      L     #T_84CLT81_READY_HIGH;
      <=R   ;
      )     ;
      U(    ;
      L     "DB_GRP_84".CLM82_HUM.PV.AV;
      L     #H_84CLM82_READY_LOW;
      >=R   ;
      )     ;
      U(    ;
      L     "DB_GRP_84".CLM82_HUM.PV.AV;
      L     #H_84CLM82_READY_HIGH;
      <=R   ;
      )     ;
      )     ;
      L     S5T#1M;
      SE    "T_CR_READY";
      NOP   0;
      NOP   0;
      NOP   0;
      U     "T_CR_READY";
      )     ;
      S     "DB_PROG_CLEAN_ROOM".CLEAN_ROOM.SM.READY;
      U(    ;
      ON    "DB_PROG_CLEAN_ROOM".CLEAN_ROOM.SM.ON;
      O(    ;
      U(    ;
      UN    "DB_POWER_SAVING_MODE2".GENERAL.SM.CR_MODE_2_ON;
      U(    ;
      ON    "DB_PROG_CLEAN_ROOM".CLEAN_ROOM.SM.TEMP_84CLT81_IN_RANGE;
      ON    "DB_PROG_CLEAN_ROOM".CLEAN_ROOM.SM.HUM_84_CLM82_IN_RANGE;
      )     ;
      O     ;
      U     "DB_POWER_SAVING_MODE2".GENERAL.SM.CR_MODE_2_ON;
      U(    ;
      O(    ;
      L     "DB_GRP_84".CLT81.PV.AV;
      L     #T_84CLT81_READY_LOW;
      <R    ;
      )     ;
      O(    ;
      L     "DB_GRP_84".CLT81.PV.AV;
      L     #T_84CLT81_READY_HIGH;
      >R    ;
      )     ;
      O(    ;
      L     "DB_GRP_84".CLM82_HUM.PV.AV;
      L     #H_84CLM82_READY_LOW;
      <R    ;
      )     ;
      O(    ;
      L     "DB_GRP_84".CLM82_HUM.PV.AV;
      L     #H_84CLM82_READY_HIGH;
      >R    ;
      )     ;
      )     ;
      )     ;
      L     S5T#1M;
      SE    "T_CR_READY_LOST_DEL";
      NOP   0;
      NOP   0;
      NOP   0;
      U     "T_CR_READY_LOST_DEL";
      )     ;
      )     ;
      R     "DB_PROG_CLEAN_ROOM".CLEAN_ROOM.SM.READY;
      NOP   0;
NETWORK
TITLE =GENERAL FAULTS
//********************************************************************************
//
//                                   GENERAL FAULTS
//
//********************************************************************************
//
// GROUP 84
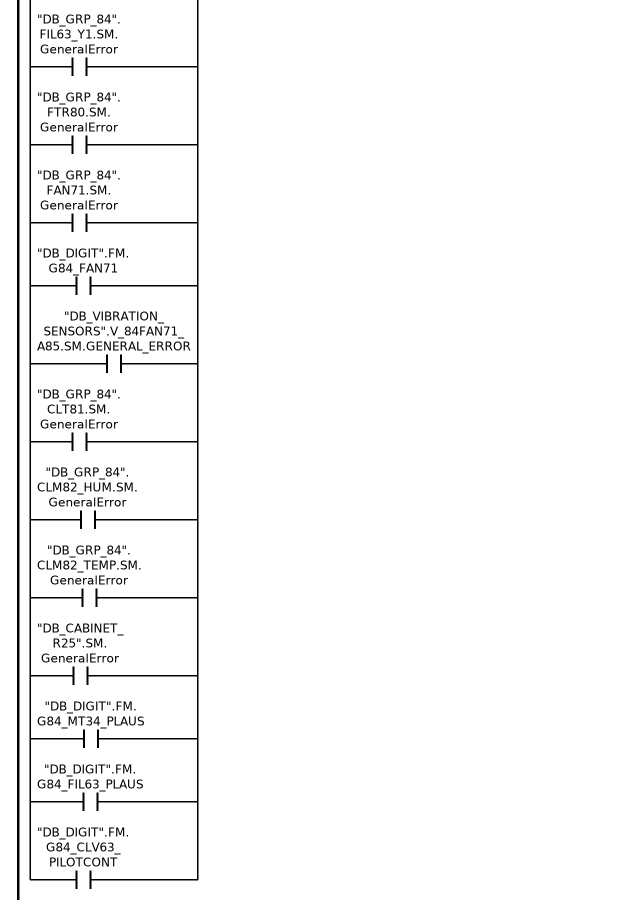
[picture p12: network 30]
      O     "DB_DIGIT".FM.G84_DOO07;
      O     "DB_GRP_84".FLA11.SM.GeneralError;
      O     "DB_GRP_84".FTR20.SM.GeneralError;
      O     "DB_GRP_84".PP30.SM.GeneralError;
      O     "DB_GRP_84".PP31.SM.GeneralError;
      O     "DB_GRP_84".VA31.SM.GeneralError;
      O     "DB_GRP_84".CLT32.SM.GeneralError;
      O     "DB_DIGIT".FM.G84_MT33;
      O     "DB_DIGIT".FM.G84_MT34_L2;
      O     "DB_GRP_84".VA41.SM.GeneralError;
      O     "DB_GRP_84".PP50.SM.GeneralError;
      O     "DB_GRP_84".PP51.SM.GeneralError;
      O     "DB_GRP_84".VA51.SM.GeneralError;
      O     "DB_DIGIT".FM.G84_MT53;
      O     "DB_GRP_84".PP61.SM.GeneralError;
      O     "DB_VIBRATION_SENSORS".V_84PP61_A85.SM.GENERAL_ERROR;
      O     "DB_DIGIT".FM.G84_FIL63_B22_1;
      O     "DB_DIGIT".FM.G84_FIL63_B21;
      O     "DB_GRP_84".FIL63_Y1.SM.GeneralError;
      O     "DB_GRP_84".FTR80.SM.GeneralError;
      O     "DB_GRP_84".FAN71.SM.GeneralError;
      O     "DB_DIGIT".FM.G84_FAN71;
      O     "DB_VIBRATION_SENSORS".V_84FAN71_A85.SM.GENERAL_ERROR;
      O     "DB_GRP_84".CLT81.SM.GeneralError;
      O     "DB_GRP_84".CLM82_HUM.SM.GeneralError;
      O     "DB_GRP_84".CLM82_TEMP.SM.GeneralError;
      O     "DB_CABINET_R25".SM.GeneralError;


      O     "DB_DIGIT".FM.G84_MT34_PLAUS;
      O     "DB_DIGIT".FM.G84_FIL63_PLAUS;
      O     "DB_DIGIT".FM.G84_CLV63_PILOTCONT;
      =     "GENERAL_FAULT_GR84";
NETWORK
TITLE =GENERAL WARNINGS
//********************************************************************************
//
//                                 GENERAL WARNINGS
//
//********************************************************************************
//
// GROUP 84
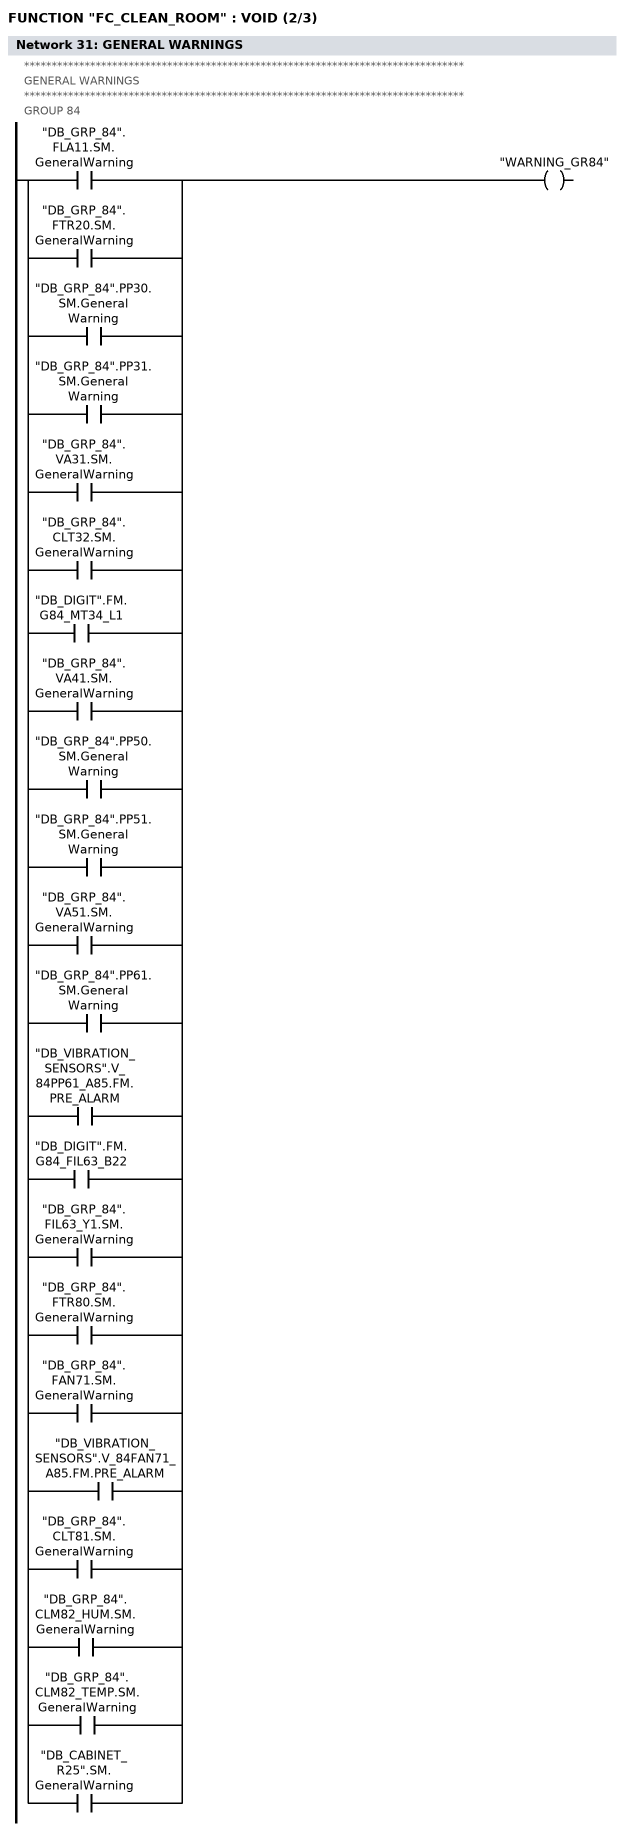
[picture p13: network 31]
      O     "DB_GRP_84".FLA11.SM.GeneralWarning;
      O     "DB_GRP_84".FTR20.SM.GeneralWarning;
      O     "DB_GRP_84".PP30.SM.GeneralWarning;
      O     "DB_GRP_84".PP31.SM.GeneralWarning;
      O     "DB_GRP_84".VA31.SM.GeneralWarning;
      O     "DB_GRP_84".CLT32.SM.GeneralWarning;
      O     "DB_DIGIT".FM.G84_MT34_L1;
      O     "DB_GRP_84".VA41.SM.GeneralWarning;
      O     "DB_GRP_84".PP50.SM.GeneralWarning;
      O     "DB_GRP_84".PP51.SM.GeneralWarning;
      O     "DB_GRP_84".VA51.SM.GeneralWarning;
      O     "DB_GRP_84".PP61.SM.GeneralWarning;
      O     "DB_VIBRATION_SENSORS".V_84PP61_A85.FM.PRE_ALARM;
      O     "DB_DIGIT".FM.G84_FIL63_B22;
      O     "DB_GRP_84".FIL63_Y1.SM.GeneralWarning;
      O     "DB_GRP_84".FTR80.SM.GeneralWarning;
      O     "DB_GRP_84".FAN71.SM.GeneralWarning;
      O     "DB_VIBRATION_SENSORS".V_84FAN71_A85.FM.PRE_ALARM;
      O     "DB_GRP_84".CLT81.SM.GeneralWarning;
      O     "DB_GRP_84".CLM82_HUM.SM.GeneralWarning;
      O     "DB_GRP_84".CLM82_TEMP.SM.GeneralWarning;
      O     "DB_CABINET_R25".SM.GeneralWarning;


      =     "WARNING_GR84";
NETWORK
TITLE =MANUAL MODE
//********************************************************************************
//
//                                   MANUAL MODE
//
//********************************************************************************
//
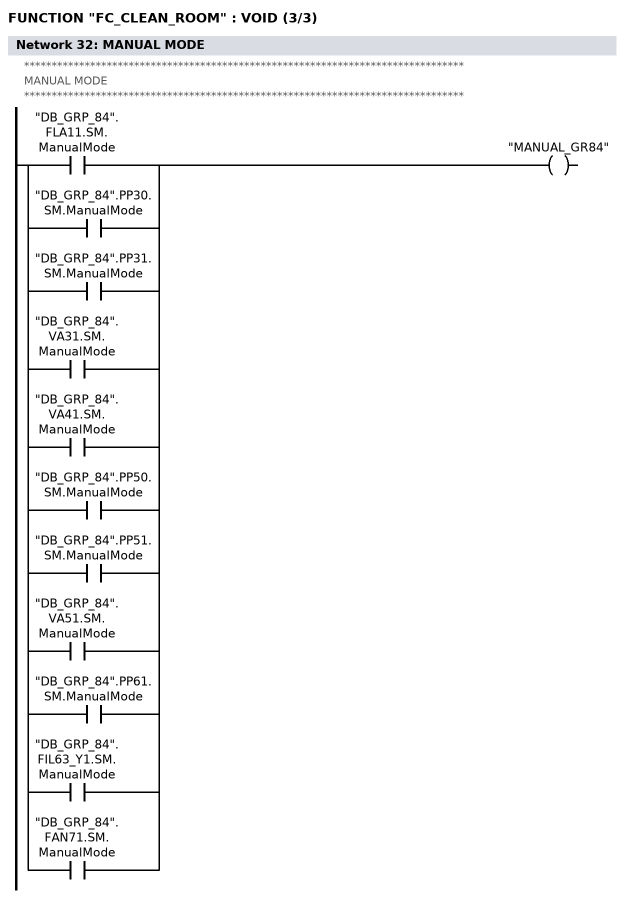
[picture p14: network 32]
      O     "DB_GRP_84".FLA11.SM.ManualMode;
      O     "DB_GRP_84".PP30.SM.ManualMode;
      O     "DB_GRP_84".PP31.SM.ManualMode;
      O     "DB_GRP_84".VA31.SM.ManualMode;
      O     "DB_GRP_84".VA41.SM.ManualMode;
      O     "DB_GRP_84".PP50.SM.ManualMode;
      O     "DB_GRP_84".PP51.SM.ManualMode;
      O     "DB_GRP_84".VA51.SM.ManualMode;
      O     "DB_GRP_84".PP61.SM.ManualMode;
      O     "DB_GRP_84".FIL63_Y1.SM.ManualMode;
      O     "DB_GRP_84".FAN71.SM.ManualMode;
      =     "MANUAL_GR84";
END_FUNCTION

